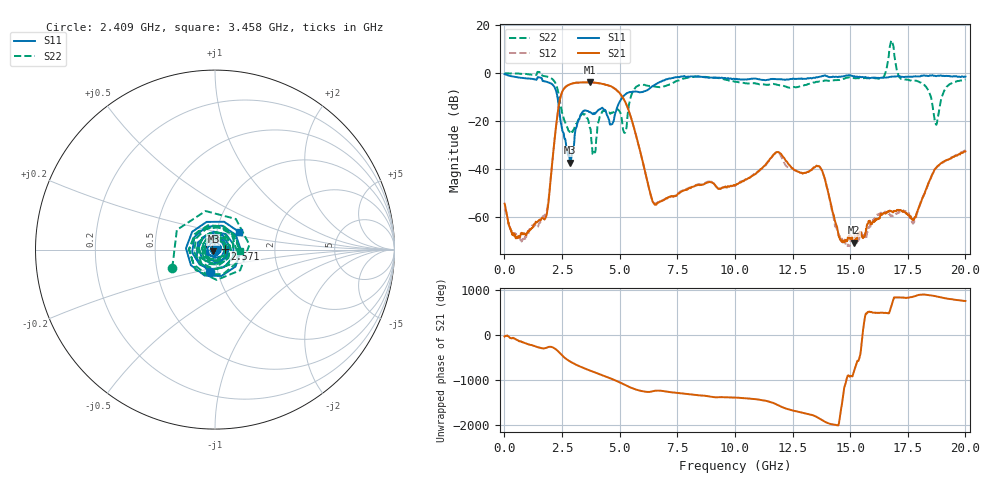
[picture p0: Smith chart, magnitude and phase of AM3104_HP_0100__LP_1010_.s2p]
!Created with skrf (http://scikit-rf.org).
# Hz S RI R 50.0
!freq ReS11 ImS11 ReS21 ImS21 ReS12 ImS12 ReS22 ImS22
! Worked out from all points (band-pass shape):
!   1601 points, 10 MHz to 20 GHz, reference 50 ohm
!   highest |S21| = -3.74 dB at 3.708 GHz (marker M1); lowest = -70.5 dB at 15.18 GHz (marker M2)
!   |S21| within 3 dB of the highest: 2.563 GHz to 4.838 GHz (2.275 GHz wide, 61.5 % of centre)
!   lowest |S11| = -37.3 dB at 2.859 GHz (marker M3), VSWR 1.03, Z = 49.1 - j1.02 ohm
!   |S11| at or under -10 dB: 2.304 GHz to 5.129 GHz (2.825 GHz wide, 76 % of centre)
!   |S22| runs from -33.9 to 13.6 dB; largest |S21 - S12| = 0.052
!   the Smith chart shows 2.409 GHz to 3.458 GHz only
!   S11 on the Smith chart (normalised r, x): 2.409 GHz: 0.91, -0.23; 2.571 GHz: 1.12, +0.01; 3.458 GHz: 1.28, +0.26
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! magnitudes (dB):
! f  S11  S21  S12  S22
! 10 MHz  -0.4  -54.3  -56.6  0.0
! 797.1 MHz  -2.0  -66.9  -69.1  -0.2
! 1.772 GHz  -3.4  -60.3  -58.9  -1.2
! 2.409 GHz  -17.8  -11.0  -11.0  -11.7
! 2.571 GHz  -25.0  -6.6  -6.6  -18.7
! 2.859 GHz  -37.3  -4.6  -4.6  -24.8
! 3.346 GHz  -16.8  -3.8  -3.9  -17.1
! 3.458 GHz  -15.6  -3.8  -3.8  -17.2
! 3.708 GHz  -16.2  -3.7  -3.8  -22.6
! 5.17 GHz  -9.5  -10.6  -10.6  -24.1
! 5.682 GHz  -7.6  -24.8  -24.9  -6.0
! 6.682 GHz  -4.0  -53.9  -53.8  -5.8
! 10.01 GHz  -2.5  -46.8  -46.8  -3.6
! 11.83 GHz  -2.5  -32.9  -32.9  -4.8
! 13.34 GHz  -2.1  -40.1  -40.1  -4.1
! 13.79 GHz  -1.1  -40.7  -40.7  -3.3
! 14.59 GHz  -1.5  -69.6  -68.1  -2.7
! 15.18 GHz  -1.2  -70.5  -66.4  -2.0
! 16.68 GHz  -1.6  -57.5  -58.6  7.2
! 17.76 GHz  -1.3  -61.0  -62.2  -3.1
! 18.73 GHz  -1.2  -39.5  -39.4  -21.4
! 20 GHz  -1.4  -32.5  -32.1  -2.6
